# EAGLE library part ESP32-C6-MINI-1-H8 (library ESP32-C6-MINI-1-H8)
8 MB (Quad SPI) , 13.2 16.6 2.4 , 3.0 ~ 3.6 V , 2.4 GHz , 2412 ~ 2484 MHz , 40C ~ 105C Source: Datasheet
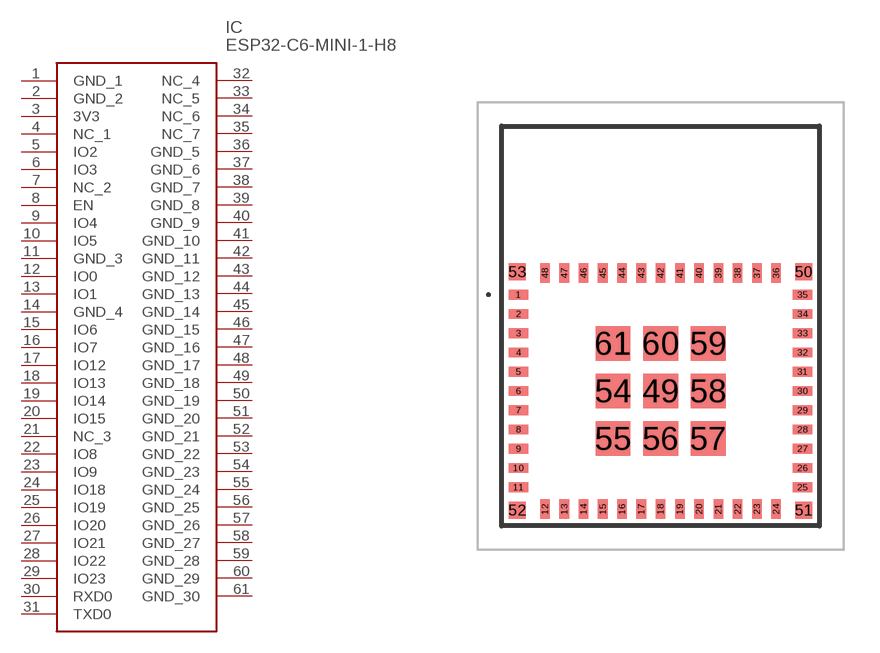
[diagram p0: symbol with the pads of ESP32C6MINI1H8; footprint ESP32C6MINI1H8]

Designator prefix IC

## ESP32-C6-MINI-1-H8 (Description: 8 MB (Quad SPI) , 13.2 16.6 2.4 , 3.0 ~ 3.6 V , 2.4 GHz , 2412 ~ 2484 MHz , 40C ~ 105C; Height: 2.55mm; Manufacturer_Name: Espressif Systems; Manufacturer_Part_Number: ESP32-C6-MINI-1-H8; Mouser_Part_Number: 356-ESP32C6MINI1H8; Mouser_Price-Stock: https://www.mouser.co.uk/ProductDetail/Espressif-Systems/ESP32-C6-MINI-1-H8?qs=olJun0bQHM8q1UR%2FHSWi2A%3D%3D)  [ESP32C6MINI1H8]
1  GND_1
2  GND_2
3  3V3
4  NC_1
5  IO2
6  IO3
7  NC_2
8  EN
9  IO4
10  IO5
11  GND_3
12  IO0
13  IO1
14  GND_4
15  IO6
16  IO7
17  IO12
18  IO13
19  IO14
20  IO15
21  NC_3
22  IO8
23  IO9
24  IO18
25  IO19
26  IO20
27  IO21
28  IO22
29  IO23
30  RXD0
31  TXD0
32  NC_4
33  NC_5
34  NC_6
35  NC_7
36  GND_5
37  GND_6
38  GND_7
39  GND_8
40  GND_9
41  GND_10
42  GND_11
43  GND_12
44  GND_13
45  GND_14
46  GND_15
47  GND_16
48  GND_17
49  GND_18
50  GND_19
51  GND_20
52  GND_21
53  GND_22
54  GND_23
55  GND_24
56  GND_25
57  GND_26
58  GND_27
59  GND_28
60  GND_29
61  GND_30

## Footprint ESP32C6MINI1H8 (pad centres in mm)
ESP32-C6-MINI-1-H8-2
smd 0.8 x 0.4: 1 -5.9,1.3; 2 -5.9,0.5; 3 -5.9,-0.3; 4 -5.9,-1.1; 5 -5.9,-1.9; 6 -5.9,-2.7; 7 -5.9,-3.5; 8 -5.9,-4.3; 9 -5.9,-5.1; 10 -5.9,-5.9; 11 -5.9,-6.7; 25 5.9,-6.7; 26 5.9,-5.9; 27 5.9,-5.1; 28 5.9,-4.3; 29 5.9,-3.5; 30 5.9,-2.7; 31 5.9,-1.9; 32 5.9,-1.1; 33 5.9,-0.3; 34 5.9,0.5; 35 5.9,1.3
smd 0.4 x 0.8: 12 -4.8,-7.6; 13 -4,-7.6; 14 -3.2,-7.6; 15 -2.4,-7.6; 16 -1.6,-7.6; 17 -0.8,-7.6; 18 0,-7.6; 19 0.8,-7.6; 20 1.6,-7.6; 21 2.4,-7.6; 22 3.2,-7.6; 23 4,-7.6; 24 4.8,-7.6; 36 4.8,2.2; 37 4,2.2; 38 3.2,2.2; 39 2.4,2.2; 40 1.6,2.2; 41 0.8,2.2; 42 0,2.2; 43 -0.8,2.2; 44 -1.6,2.2; 45 -2.4,2.2; 46 -3.2,2.2; 47 -4,2.2; 48 -4.8,2.2
smd 1.45 x 1.45: 49 0,-2.7; 54 -1.975,-2.7; 55 -1.975,-4.675; 56 0,-4.675; 57 1.975,-4.675; 58 1.975,-2.7; 59 1.975,-0.725; 60 0,-0.725; 61 -1.975,-0.725
smd 0.7 x 0.7: 50 5.95,2.25; 51 5.95,-7.65; 52 -5.95,-7.65; 53 -5.95,2.25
